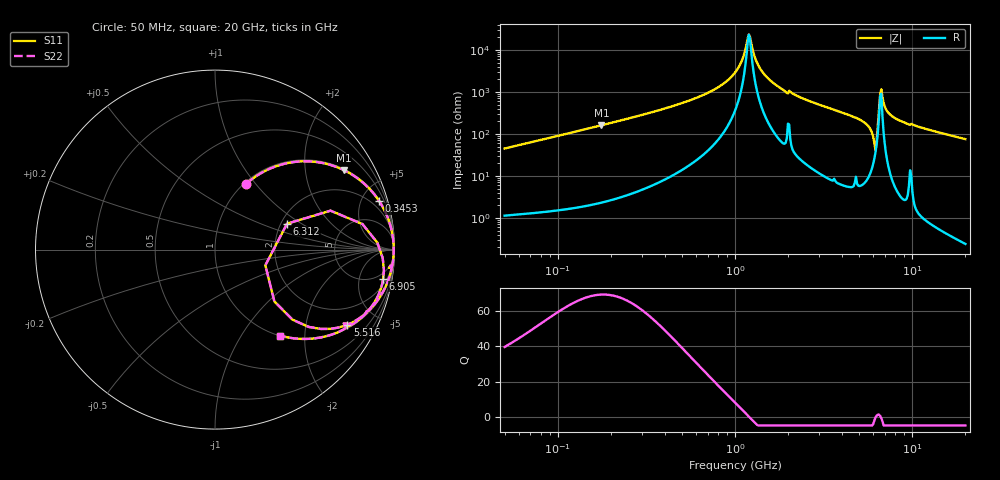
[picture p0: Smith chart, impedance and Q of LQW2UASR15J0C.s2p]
!Murata Part Number: LQW2UASR15J0C
!These Parameters are Measured in Series Mode Connection
!  o--[Z]--o
!Port1  Port2
!  o-------o
!Freq. Start=50[MHz] Stop=20[GHz], 401[Steps]
# Hz S RI R 50
!Freq.(Hz) S11(Real) S11(Imag) S21(Real) S21(Imag) S12(Real) S12(Imag) S22(Real) S22(Imag)
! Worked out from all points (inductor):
!   401 points, 50 MHz to 20 GHz, reference 50 ohm
!   read as one part in series: L = 143 nH near 51.52 MHz
!   highest Q = 69.6 at 176 MHz (marker M1), where L = 145 nH
!   self-resonance near 1.197 GHz
!   S11 on the Smith chart (normalised r, x): 50 MHz: 1.02, +0.90; 345.3 MHz: 1.12, +6.72; 5.516 GHz: 1.15, -3.43; 6.312 GHz: 2.16, +0.76; 6.905 GHz: 3, -11; 20 GHz: 1.00, -1.50
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5e7  0.1744 0.3671  0.8256 -0.3671  0.8256 -0.3671  0.1744 0.3671
1.364002e8  0.6024 0.482  0.3976 -0.482  0.3976 -0.482  0.6024 0.482
1.759554e8  0.7178 0.443  0.2822 -0.443  0.2822 -0.443  0.7178 0.443
3.452505e8  0.9145 0.2708  0.0855 -0.2708  0.0855 -0.2708  0.9145 0.2708
3.721004e8  0.9269 0.251  0.0731 -0.251  0.0731 -0.251  0.9269 0.251
7.08568e8  0.9852 0.1012  0.0148 -0.1012  0.0148 -0.1012  0.9852 0.1012
1e9  0.9946 0.034  0.00542 -0.034  0.00542 -0.034  0.9946 0.034
1.094034e9  0.9955 0.0172  0.00454 -0.0172  0.00454 -0.0172  0.9955 0.0172
1.196911e9  0.9958 0.000458  0.00423 -0.000458  0.00423 -0.000458  0.9958 0.000458
1.349283e9  0.9953 -0.022  0.00472 0.022  0.00472 0.022  0.9953 -0.022
1.544007e9  0.9934 -0.0478  0.00655 0.0478  0.00655 0.0478  0.9934 -0.0478
1.932977e9  0.9846 -0.0965  0.0154 0.0965  0.0154 0.0965  0.9846 -0.0965
2.728004e9  0.9663 -0.168  0.0337 0.168  0.0337 0.168  0.9663 -0.168
5.515528e9  0.7371 -0.4185  0.2629 0.4185  0.2629 0.4185  0.7371 -0.4185
5.944466e9  0.5212 -0.4305  0.4788 0.4305  0.4788 0.4305  0.5212 -0.4305
6.125241e9  0.3306 -0.2883  0.6694 0.2883  0.6694 0.2883  0.3306 -0.2883
6.311513e9  0.401 0.144  0.599 -0.144  0.599 -0.144  0.401 0.144
6.601595e9  0.9042 0.0391  0.0958 -0.0391  0.0958 -0.0391  0.9042 0.0391
6.905011e9  0.9374 -0.1614  0.0626 0.1614  0.0626 0.1614  0.9374 -0.1614
7.442007e9  0.8899 -0.2915  0.1101 0.2915  0.1101 0.2915  0.8899 -0.2915
9.316812e9  0.7558 -0.4216  0.2442 0.4216  0.2442 0.4216  0.7558 -0.4216
2e10  0.3612 -0.4788  0.6388 0.4788  0.6388 0.4788  0.3612 -0.4788
